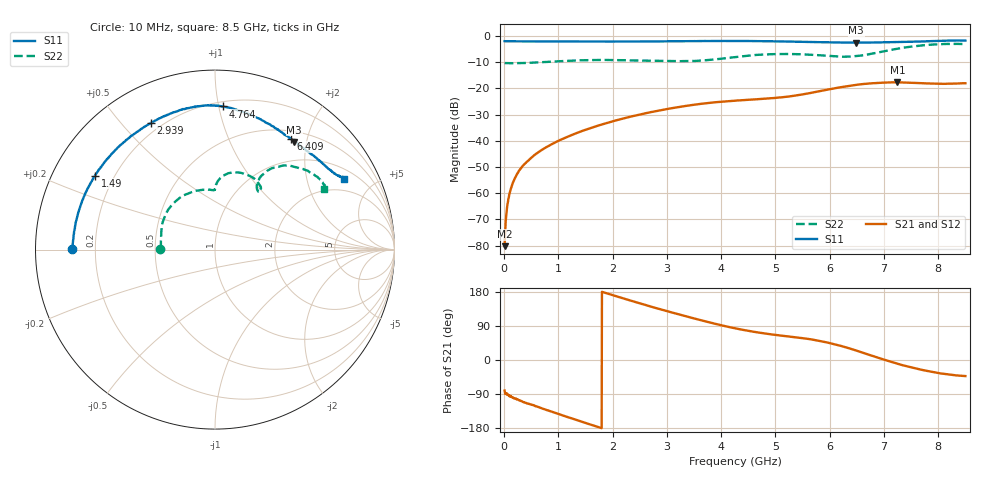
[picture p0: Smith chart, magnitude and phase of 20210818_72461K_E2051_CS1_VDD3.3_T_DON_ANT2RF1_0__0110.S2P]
!Agilent Technologies,E5071C,MY46417908,A.11.23
!Date: Wed Aug 18 14:23:36 2021
!Data & Calibration Information:
!Freq	S11:SOLT2(ON)	S21:SOLT2(ON)	S12:SOLT2(ON)	S22:SOLT2(ON)
!PortZ  Port1:50+j0  Port2:50+j0
!Above PortZ is port z conversion or system Z0 setting when saving the data.
!When reading, reference impedance value at option line is always used.
# Hz S dB R 50
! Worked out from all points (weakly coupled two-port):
!   1601 points, 10 MHz to 8.5 GHz, reference 50 ohm
!   highest |S21| = -17.67 dB at 7.248 GHz (marker M1); lowest = -80.2 dB at 10 MHz (marker M2)
!   lowest |S11| = -2.6 dB at 6.489 GHz (marker M3), VSWR 6.85, Z = 33.1 + j89.3 ohm
!   |S11| at or under -10 dB: nowhere
!   |S22| runs from -10.4 to -3.0 dB; largest |S21 - S12| = 0.00065
!   S11 on the Smith chart (normalised r, x): 10 MHz: 0.11, +0.00; 1.49 GHz: 0.13, +0.28; 2.939 GHz: 0.16, +0.60; 4.764 GHz: 0.23, +1.03; 6.409 GHz: 0.62, +1.73; 8.5 GHz: 1.39, +3.34
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1e7  -1.97 179.7  -80.21 -80.6  -79.44 -73.0  -10.32 179.6
6.836875e7  -2.01 178.6  -63.62 -91.9  -63.79 -91.5  -10.35 178.1
1.108188e8  -2.01 177.6  -59.40 -95.4  -59.45 -95.2  -10.36 176.9
1.957188e8  -2.03 175.8  -54.40 -101.1  -54.46 -101.3  -10.38 174.4
3.124562e8  -2.04 173.3  -50.39 -107.8  -50.42 -108.4  -10.33 171.6
5.140938e8  -2.04 169.2  -46.29 -117.9  -46.28 -118.0  -10.21 166.5
7.210375e8  -2.06 164.7  -43.13 -128.7  -43.13 -128.9  -9.98 160.5
1.426769e9  -2.09 149.7  -36.33 -162.6  -36.35 -162.6  -9.26 136.4
1.490444e9  -2.10 148.4  -35.88 -165.7  -35.88 -165.6  -9.23 134.1
2.164338e9  -2.10 133.6  -31.64 164.0  -31.65 164.0  -9.22 110.8
2.843538e9  -2.05 118.9  -28.50 135.4  -28.50 135.3  -9.50 95.0
2.93905e9  -2.04 117.0  -28.12 131.7  -28.11 131.7  -9.56 93.7
3.565188e9  -1.95 105.1  -26.06 107.3  -26.05 107.3  -9.47 90.1
4.255e9  -1.89 94.2  -24.68 83.7  -24.68 83.7  -8.04 86.1
4.7644e9  -1.95 86.9  -23.98 70.8  -23.98 70.9  -7.08 76.2
5.671769e9  -2.28 70.9  -21.64 54.1  -21.66 54.2  -7.20 55.2
6.409338e9  -2.51 55.5  -18.85 28.6  -18.88 28.5  -7.77 54.6
6.488931e9  -2.55 53.6  -18.66 25.0  -18.69 24.9  -7.68 55.6
7.088538e9  -2.37 42.1  -17.72 -2.8  -17.75 -3.0  -5.43 56.0
7.247725e9  -2.30 39.5  -17.67 -9.8  -17.69 -9.8  -4.84 53.4
8.001212e9  -1.88 30.3  -18.21 -34.4  -18.20 -34.4  -3.15 36.1
8.5e9  -1.74 28.9  -18.02 -42.4  -18.03 -42.6  -3.13 29.2
